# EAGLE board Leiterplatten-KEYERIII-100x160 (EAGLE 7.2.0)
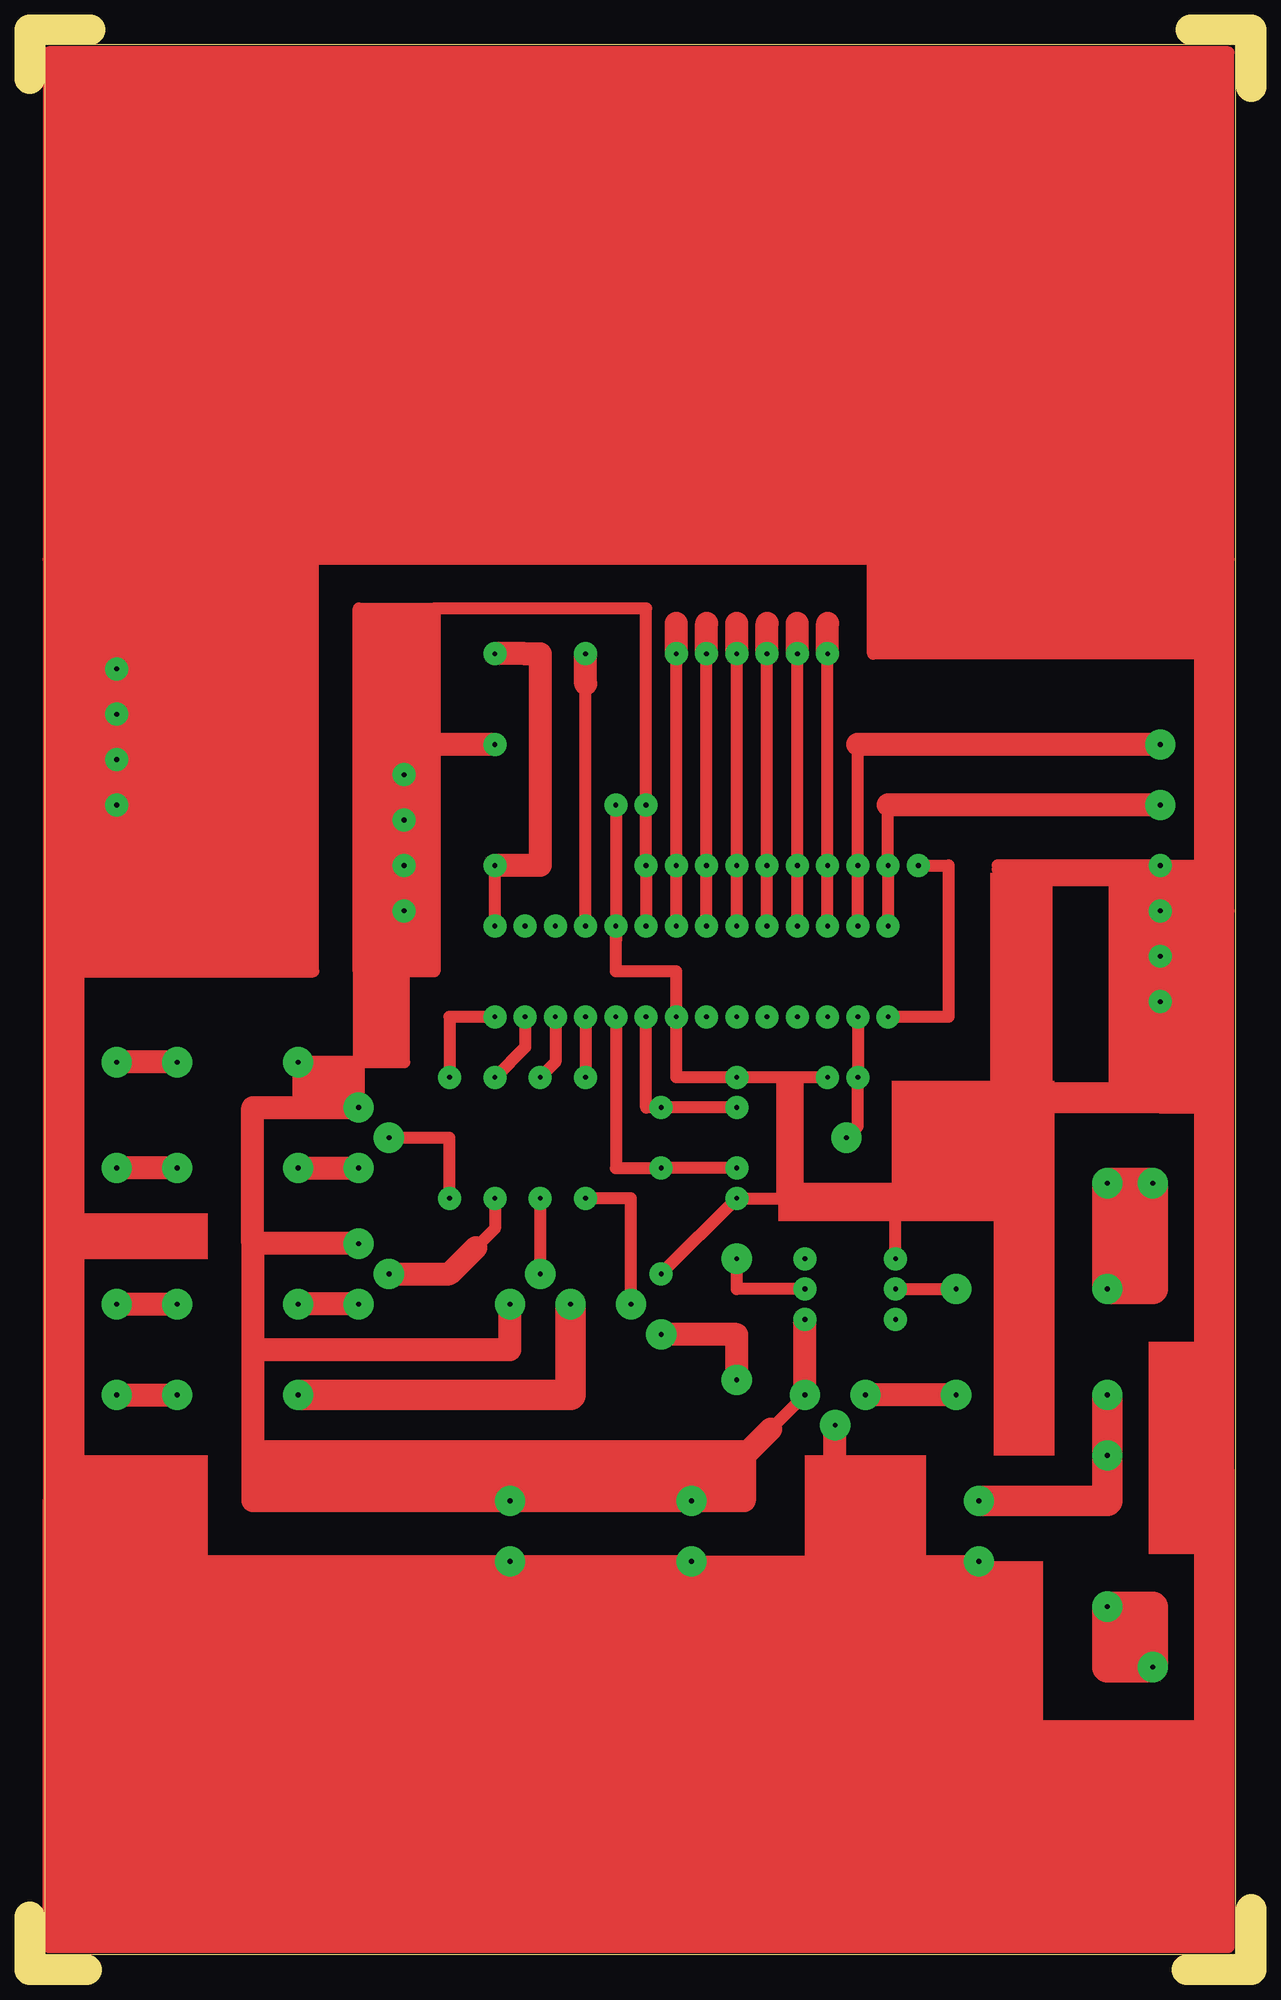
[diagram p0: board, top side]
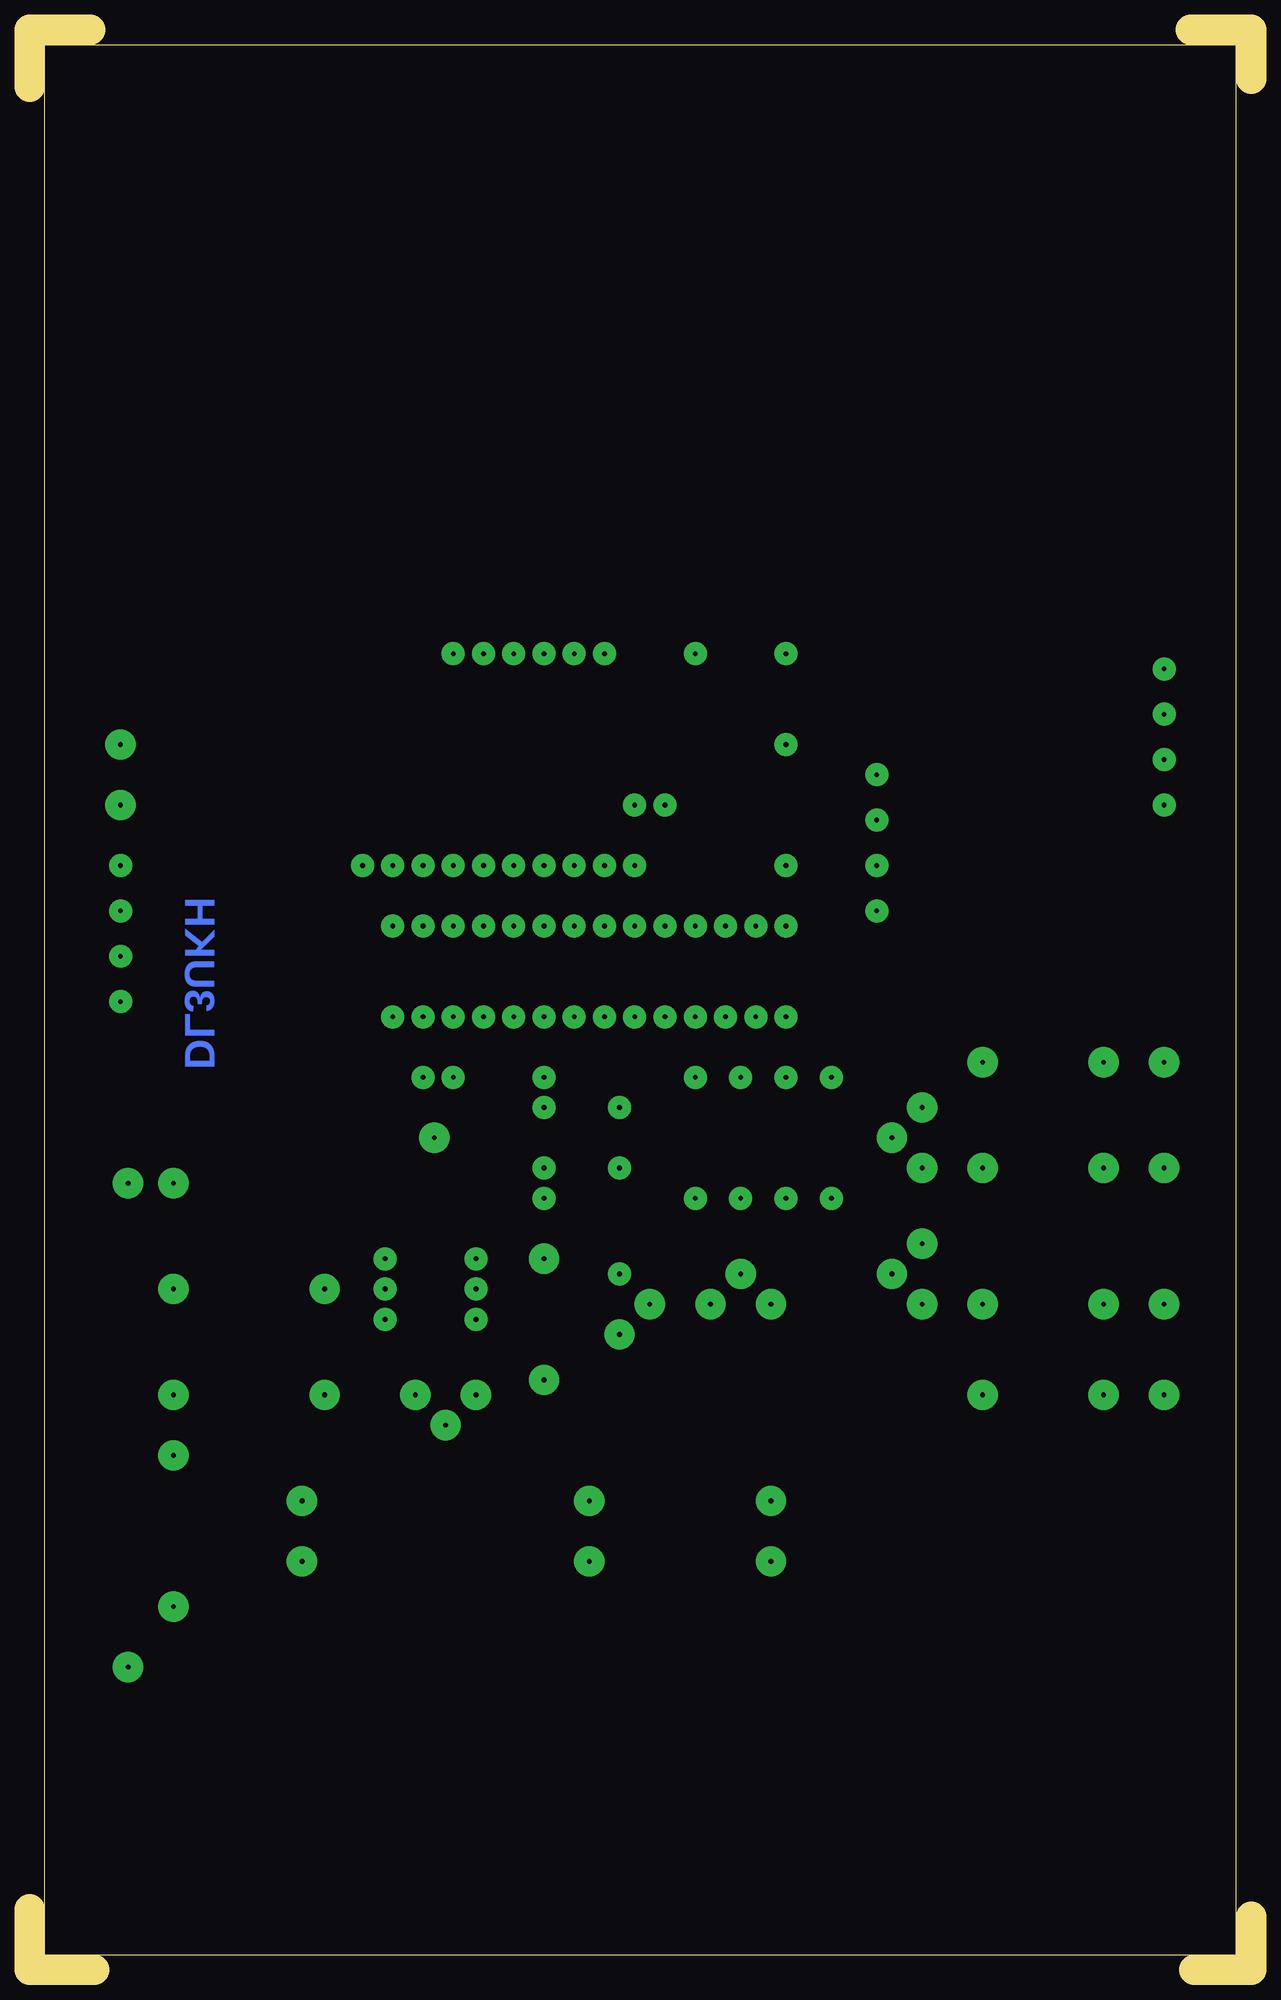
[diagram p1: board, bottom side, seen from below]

Size 102.55 x 162.88 mm. Coordinates in mm from the lower left corner, seen from the top.
Outline: 97.16,0 102.23,0
Outline: 102.55,0 102.55,5.08
Outline: 4.76,0 0,0 0,4.45
Outline: 97.47,162.88 102.55,162.88 102.55,158.11
Outline: 0,158.75 0,162.88
Outline: 5.08,162.88 0.32,162.88
Outline: 101.28,1.27 1.27,1.27 1.27,161.61 101.28,161.61 101.28,1.27
Copper layers (1*16): Top 0.035mm / dielectric 1.5mm / Bottom 0.035mm
Design rules "default": minimum track width 10mil, minimum drill 24mil, track to track 8mil, track to pad 8mil, pad to pad 8mil, via to via 8mil, smd to smd 8mil, copper to edge 40mil, drill to drill 8mil, minimum pad ring 10mil, minimum via ring 8mil, stop-mask expansion 4mil, vias tented up to drill 0mil, thermal gap 10mil

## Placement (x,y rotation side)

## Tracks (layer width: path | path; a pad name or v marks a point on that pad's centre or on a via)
S$1  (via drill 0.4 pad 1.93)
  Top 1.016: v39.05,80.01 35.24,80.01 v35.24,74.93
S$2  (via drill 0.4 pad 1.93)
  other vias: 41.59,80.01
S$3  (via drill 0.4 pad 1.93)
  Top 1.016: v44.13,80.01 44.13,76.2 v42.86,74.93
S$4  (via drill 0.4 pad 1.93)
  Top 1.016: v46.67,80.01 v46.67,74.93
S$5  (via drill 0.4 pad 1.93, 0.4 pad 2.54)
  Top 1.016: v50.48,55.88 50.48,64.77 v46.67,64.77
S$6  (via drill 0.4 pad 1.93, 0.4 pad 2.54)
  Top 1.016: v42.86,64.77 v42.86,58.42
S$7  (via drill 0.4 pad 1.93)
  Top 1.016: 41.59,79.69 41.59,77.47 v39.05,74.93
S$8  (via drill 0.4 pad 1.93)
  other vias: 56.83,80.01
S$9  (via drill 0.4 pad 1.93)
  other vias: 59.37,80.01
S$10  (via drill 0.4 pad 1.93)
  other vias: 61.91,80.01
S$11  (via drill 0.4 pad 1.93)
  other vias: 64.45,80.01
S$12  (via drill 0.4 pad 1.93)
  other vias: 66.99,80.01
S$13  (via drill 0.4 pad 1.93)
  other vias: 31.43,88.9
S$14  (via drill 0.4 pad 2.54)
  Top 1.016: v22.54,48.26 40,48.26 | 45.4,53.66 v45.4,55.88
  Top 2.54: v22.54,48.26 45.4,48.26 v45.4,55.88
S$15  (via drill 0.4 pad 1.93)
  Top 1.016: v39.05,87.63 39.05,92.71 | 41.59,110.49 v39.05,110.49
  Top 1.93: 41.59,110.49 42.86,110.49 42.86,92.71 39.05,92.71
S$16  (via drill 0.4 pad 1.93)
  other vias: 41.59,87.63
S$17  (via drill 0.4 pad 1.93)
  other vias: 44.13,87.63
S$18  (via drill 0.4 pad 1.93)
  Top 1.016: v46.67,87.63 46.67,110.49
S$19  (via drill 0.4 pad 1.93)
  Top 1.016: v59.37,72.39 v53.02,72.39 51.75,72.39 v51.75,80.01
S$20  (via drill 0.4 pad 1.93)
  other vias: 46.67,110.49
S$21  (via drill 0.4 pad 1.93)
  other vias: 54.29,87.63
S$22  (via drill 0.4 pad 1.93)
  other vias: 56.83,87.63
S$23  (via drill 0.4 pad 1.93)
  other vias: 59.37,87.63
S$24  (via drill 0.4 pad 1.93)
  other vias: 61.91,87.63
S$25  (via drill 0.4 pad 1.93)
  other vias: 64.45,87.63
S$26  (via drill 0.4 pad 1.93)
  other vias: 66.99,87.63
S$27  (via drill 0.4 pad 1.93)
  other vias: 69.53,87.63
S$28  (via drill 0.4 pad 1.93)
  Top 1.016: v49.21,80.01 49.21,67.31 v53.02,67.31 v59.37,67.31
S$29  (via drill 0.4 pad 1.93)
  other vias: 7.3,97.79
S$30  (via drill 0.4 pad 1.93)
  other vias: 31.43,96.52
S$31  (via drill 0.4 pad 1.93, 0.4 pad 2.54)
  Top 1.016: v69.53,92.71 69.53,102.87
  Top 1.93: v94.93,102.87 69.53,102.87
S$32  (via drill 0.4 pad 1.93)
  other vias: 66.99,92.71
S$33  (via drill 0.4 pad 1.93)
  other vias: 64.45,92.71
S$34  (via drill 0.4 pad 1.93)
  other vias: 61.91,92.71
S$35  (via drill 0.4 pad 1.93)
  other vias: 59.37,92.71
S$36  (via drill 0.4 pad 1.93)
  other vias: 56.83,92.71
S$37  (via drill 0.4 pad 1.93)
  other vias: 54.29,92.71
S$38  (via drill 0.4 pad 2.54)
  Top 1.93: v7.3,48.26 v12.38,48.26
S$39  (via drill 0.4 pad 1.93, 0.4 pad 2.54)
  Top 1.016: v35.24,64.77 35.24,69.85 v30.16,69.85
S$40  (via drill 0.4 pad 2.54)
  Top 1.016: v90.49,66.04 90.49,66.36
  Top 2.54: v90.49,57.15 v90.49,66.04 v94.3,66.04 94.3,57.15 v90.49,57.15
S$41  (via drill 0.4 pad 1.93)
  Top 1.93: v66.99,110.49 66.99,113.03 | 64.45,110.49 64.45,113.03 | 61.91,110.49 61.91,113.03 | 59.37,110.49 59.37,113.03 | 56.83,110.49 56.83,113.03 | 54.29,110.49 54.29,113.03 | 46.67,107.95 46.67,110.49 | 41.59,110.49 39.05,110.49
S$42  (via drill 0.4 pad 1.93)
  other vias: 64.45,110.49
S$43  (via drill 0.4 pad 1.93)
  other vias: 61.91,110.49
S$44  (via drill 0.4 pad 1.93)
  other vias: 59.37,110.49
S$45  (via drill 0.4 pad 1.93)
  other vias: 56.83,110.49
S$46  (via drill 0.4 pad 1.93)
  other vias: 54.29,110.49
S$47  (via drill 0.4 pad 1.93)
  other vias: 59.37,74.93
S$48  (via drill 0.4 pad 2.54)
  Top 1.93: v22.54,67.31 v27.62,67.31
S$49  (via drill 0.4 pad 1.93)
  other vias: 7.3,101.6
S$50  (via drill 0.4 pad 1.93)
  other vias: 31.43,100.33
S$51  (via drill 0.4 pad 1.93, 0.4 pad 2.54)
  Top 1.016: v72.07,87.63 v72.07,92.71 72.07,97.79 | 69.53,87.63 v69.53,92.71 | 66.99,87.63 66.99,110.49 | 64.45,87.63 64.45,110.49 | 61.91,87.63 61.91,110.49 | 59.37,87.63 59.37,110.49 | 56.83,87.63 56.83,110.49 | 54.29,87.63 54.29,110.49
  Top 1.93: v94.93,97.79 72.07,97.79
S$52  (via drill 0.4 pad 1.93)
  other vias: 7.3,105.41
S$53  (via drill 0.4 pad 2.54)
  Top 1.93: v27.62,55.88 v22.54,55.88
S$56  (via drill 0.4 pad 1.93)
  other vias: 39.05,92.71
S$57  (via drill 0.4 pad 2.54)
  Top 1.93: v12.38,76.2 v7.3,76.2
S$58  (via drill 0.4 pad 1.93)
  other vias: 94.93,88.9
S$59  (via drill 0.4 pad 2.54)
  Top 1.93: v12.38,67.31 v7.3,67.31
S$60  (via drill 0.4 pad 1.93, 0.4 pad 2.54)
  Top 1.016: v72.71,57.15 v77.79,57.15
S$61  (via drill 0.4 pad 2.54)
  Top 1.93: v7.3,55.88 v12.38,55.88
S$62  (via drill 0.4 pad 1.93)
  other vias: 7.3,109.22
S$63
  Top 1.016: 94.62,92.71 91.12,92.71 | 91.12,92.71 81.28,92.71 | 91.12,72.71 91.12,73.98 | 91.12,73.98 91.12,91.44 | 91.12,91.44 91.12,92.71 | 85.41,72.71 85.41,73.98 | 85.41,73.98 85.41,91.44 | 85.41,91.44 85.41,92.39 81.28,92.39 | 91.12,73.98 85.41,73.98 | 91.12,91.44 85.41,91.44
S$64  (via drill 0.4 pad 2.54)
  Top 1.93: v77.79,48.26 v70.17,48.26
S$65  (via drill 0.4 pad 1.93)
  other vias: 31.43,92.71
S$66
  Top 1.93: 67.63,31.75 67.63,46.04
S$67  (via drill 0.4 pad 2.54)
  Top 1.93: v90.49,48.26 v90.49,43.18 90.49,39.37
  Top 2.54: v79.69,39.37 90.49,39.37 v90.49,48.26
S$68  (via drill 0.4 pad 2.54)
  Top 2.54: v94.3,25.4 94.3,30.48 v90.49,30.48 90.49,25.4 v94.3,25.4
S$69  (via drill 0.4 pad 1.93, 0.4 pad 2.54)
  Top 1.016: v69.53,80.01 v69.53,74.93 69.53,70.8 v68.58,69.85
S$70  (via drill 0.4 pad 1.93, 0.4 pad 2.54)
  Top 1.016: 19.37,60.96 18.73,60.96 | v51.75,87.63 v51.75,92.71 v51.75,97.79 51.75,114.3 33.97,114.3 | 33.97,114.3 33.97,102.87 | 33.97,102.87 33.97,83.82 31.43,83.82 | 34.29,102.87 33.97,102.87 | 31.43,83.82 27.62,83.82 | 27.62,83.82 27.62,76.2 | 27.62,76.2 v27.62,72.39 | 27.62,76.2 v22.54,76.2 22.54,72.39 | 27.62,83.82 27.62,114.3 33.97,114.3 | 27.62,76.2 31.43,76.2 31.43,83.82 | v65.09,48.26 62.23,45.4
  Top 1.93: v65.09,48.26 v65.09,54.61 | v27.62,72.39 22.54,72.39 18.73,72.39 18.73,60.96 18.73,52.07 | 18.73,52.07 40.32,52.07 v40.32,55.88 | 18.73,52.07 18.73,39.37 v40.32,39.37 v55.56,39.37 60.01,39.37 60.01,43.18 | v39.05,102.87 34.29,102.87 | v27.62,60.96 19.37,60.96 | 60.01,43.18 62.23,45.4 | 60.01,43.18 60.01,43.5 19.05,43.5
S$71
  Top 1.93: 81.6,73.03 72.71,64.13
S$72  (via drill 0.4 pad 1.93)
  Top 1.016: v72.07,80.01 77.15,80.01 77.15,92.71 v74.61,92.71
S$73  (via drill 0.4 pad 2.54)
  Top 1.016: 67.63,34.29 v55.56,34.29 v40.32,34.29 2.22,34.29 | v67.63,45.72 67.63,34.29 | v79.69,34.29 67.63,34.29
S$74  (via drill 0.4 pad 1.93)
  Top 1.016: 94.93,88.9 v94.93,92.71 99.06,92.71 | 94.93,88.9 v94.93,85.09 | 100.65,41.91 100.65,88.9 | 100.65,88.9 94.93,88.9 | 100.65,88.9 100.65,118.43 | 100.65,118.43 23.81,118.43 | 23.81,118.43 1.59,118.43 | 1.59,118.43 1.59,39.37 | 1.59,39.37 4.13,18.1 4.13,83.82 23.81,83.82 23.81,118.43 | 100.65,41.91 99.38,2.22 99.38,72.39 | 100.65,41.91 100.65,1.91 1.91,1.91 | 1.91,14.92 1.91,1.91 | 1.91,1.91 1.59,1.91 1.59,39.37 | 100.65,118.43 100.65,160.97 1.59,160.97 1.59,118.43 | 95.25,85.09 v94.93,85.09 | 80.96,72.71 80.96,72.39 | 80.96,72.39 73.34,64.77 64.45,64.77 | v49.21,87.63 49.21,86.36 | v49.21,87.63 49.21,83.82 54.29,83.82 v54.29,80.01 54.29,74.93 64.45,74.93 | v49.21,97.79 v49.21,87.63 | v66.99,74.93 64.45,74.93 | 64.45,74.93 64.45,64.77 | 63.18,64.77 v59.37,64.77 v53.02,58.42 | 63.18,64.77 64.45,64.77 | v94.93,85.09 v94.93,81.28 94.93,72.39 | 94.93,72.39 80.96,72.39 | 99.38,72.39 99.38,110.49 | 99.38,110.49 98.74,122.24 | 94.93,72.39 99.38,72.39 | 99.38,110.49 70.8,110.49 70.8,118.75 | 63.18,64.77 63.18,74.61
S$75  (via drill 0.4 pad 1.93)
  other vias: 72.71,54.61
S$76  (via drill 0.4 pad 1.93)
  Top 1.016: v72.71,59.69 72.71,64.45
S$77  (via drill 0.4 pad 1.93)
  other vias: 65.09,59.69
S$78  (via drill 0.4 pad 1.93, 0.4 pad 2.54)
  Top 1.016: v65.09,57.15 59.37,57.15 v59.37,59.69
S$79  (via drill 0.4 pad 1.93, 0.4 pad 2.54)
  Top 1.016: v39.05,64.77 39.05,62.23 37.46,60.64 | v30.16,58.42 35.24,58.42
  Top 1.93: 29.85,58.42 35.24,58.42 37.46,60.64
S$80  (via drill 0.4 pad 2.54)
  Top 1.016: v53.02,53.34 52.7,53.34
  Top 1.93: v59.37,49.53 59.37,53.34 v53.02,53.34
(copper drawn outside any net)
  shapes: Top area x32

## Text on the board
Bottom: DL3UKH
